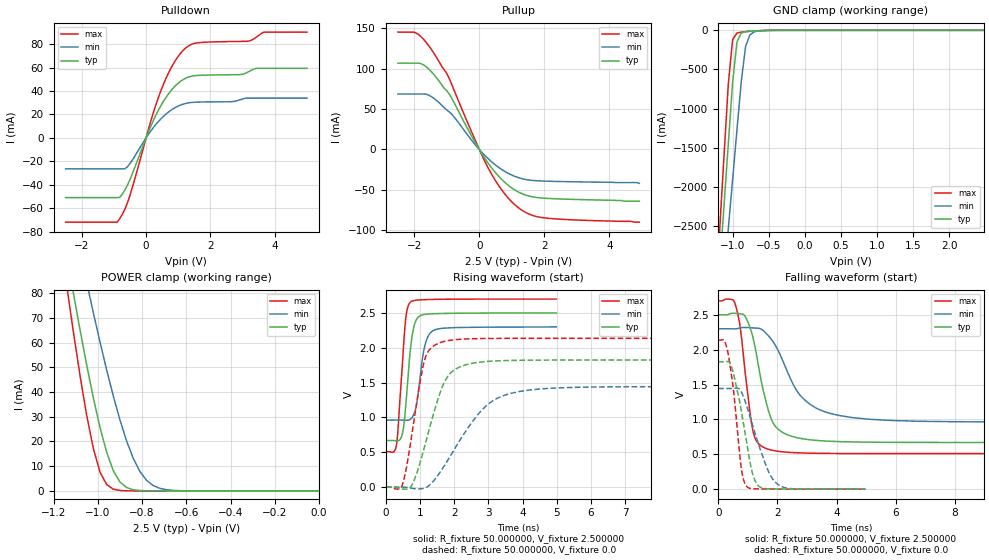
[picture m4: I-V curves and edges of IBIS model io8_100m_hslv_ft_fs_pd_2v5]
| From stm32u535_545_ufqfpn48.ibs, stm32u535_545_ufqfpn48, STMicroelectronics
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|   Model io8_100m_hslv_ft_fs_pd_2v5
[Model]  io8_100m_hslv_ft_fs_pd_2v5
Model_type I/O
Polarity   Non-Inverting
Enable   Active-Low
Vinl =   0.750000V
Vinh =   1.750000V
Vmeas =  1.250000V
Cref =   50.000000pF
Rref =   100.000000M
Vref =   0.0V
C_comp   3.340900pF   3.338500pF   3.380300pF
[Temperature Range]   25.000000   0.140000k   -40.000000
[Pullup Reference]   2.500000V   2.300000V   2.700000V
[Pulldown Reference]   0.0V   0.0V   0.0V
[POWER Clamp Reference]   2.500000V   2.300000V   2.700000V
[GND Clamp Reference]   0.0V   0.0V   0.0V
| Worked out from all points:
|   slope of the pulldown table from 0 to 0.375 V, typ, clamps not added: 16.1 ohm
|   slope of the pullup table from 0 to 0.375 V, typ, clamps not added: 16.6 ohm
|   GND clamp passes 1 mA (typ) near -0.50 V on its own axis
|   POWER clamp passes 1 mA (typ) near -0.86 V on its own axis
|   rising waveform, R_fixture 50.000000, V_fixture 2.500000: 20-80 % time 200ps typ, 231ps min, 180ps max; typ from 0.67 V to 2.5 V
|   rising waveform, R_fixture 50.000000, V_fixture 0.0: 20-80 % time 660ps typ, 1.22ns min, 424ps max; typ from 0 V to 1.82 V
|   falling waveform, R_fixture 50.000000, V_fixture 2.500000: 20-80 % time 569ps typ, 1.09ns min, 362ps max; typ from 2.5 V to 0.67 V
|   falling waveform, R_fixture 50.000000, V_fixture 0.0: 20-80 % time 467ps typ, 671ps min, 321ps max; typ from 1.82 V to 0 V
[Pulldown]
|Voltage   I(typ)   I(min)   I(max)
-2.5V     -51.01mA   -26.45mA   -72.04mA
-900mV    -51.01mA   -26.45mA   -72.04mA
-820mV    -50.89mA   -26.45mA   -69.09mA
-500mV    -35.59mA   -21.93mA   -49.09mA
140mV     9.489mA    5.639mA    13.76mA
460mV     27.5mA     16.25mA    40.22mA
860mV     43.07mA    25.18mA    63.88mA
1.26V     51.38mA    29.65mA    77.49mA
1.66V     53.45mA    30.63mA    81.42mA
3.18V     56.44mA    34.01mA    82.68mA
3.66V     59.44mA    34.01mA    90.42mA
5V        59.44mA    34.01mA    90.42mA
[Pullup]
|Voltage   I(typ)   I(min)   I(max)
-2.5V     106.7mA    68.56mA    145.2mA
-1.96V    106.7mA    68.56mA    144.4mA
-1.72V    104.8mA    68.56mA    136.6mA
-1.48V    96.52mA    65.55mA    124.2mA
-1V       72.68mA    48.88mA    94.22mA
-120mV    8.307mA    5.657mA    10.97mA
280mV     -17.4mA    -11.68mA   -23.32mA
680mV     -36.72mA   -24.56mA   -49.54mA
1.16V     -51.75mA   -34.32mA   -70.71mA
1.56V     -58mA      -38.01mA   -80.45mA
1.96V     -60.18mA   -39.11mA   -84.44mA
4.92V     -64mA      -42mA      -90mA
[GND_clamp]
|Voltage   I(typ)   I(min)   I(max)
-2.5V     -9.446A    -9.524A    -9.146A
-1.18V    -3.045A    -3.8A      -2.552A
-1.12V    -2.248A    -3.166A    -1.614A
-1.06V    -1.452A    -2.533A    -685.4mA
-1V       -665mA     -1.901A    -117.9mA
-940mV    -148mA     -1.272A    -34.34mA
-880mV    -35.14mA   -651.5mA   -22.8mA
-820mV    -16.02mA   -203.9mA   -17.08mA
-760mV    -10.47mA   -56.89mA   -12.28mA
-700mV    -7.079mA   -18.53mA   -8.16mA
-400mV    -112.4uA   -382.5uA   -53.84uA
2.48V     63.1uA     48.03uA    77.39uA
[POWER_clamp]
|Voltage   I(typ)   I(min)   I(max)
-2.49V    881mA      773.1mA    1.07A
-1.14V    95.25mA    122.7mA    82.82mA
-1.11V    79.9mA     109.7mA    64.14mA
-1.05V    50.87mA    84.26mA    30.57mA
-1.02V    37.63mA    72.04mA    17.17mA
-990mV    25.71mA    60.25mA    7.621mA
-930mV    8.217mA    38.43mA    713.9uA
-900mV    3.624mA    28.77mA    182.8uA
-840mV    490.7uA    13.24mA    11.35uA
-780mV    56.55uA    4.324mA    699nA
-660mV    716.5nA    226uA      9.775nA
0V        0A         19.49nA    0A
[Ramp]
| variable   typ   min   max
dV/dt_r  1.09464/0.65908n   0.86550/1.21773n   1.28148/0.42322n
dV/dt_f  1.09787/0.56785n   0.80201/1.08800n   1.31323/0.36140n
R_load = 50.000000
[Rising Waveform]
R_fixture= 50.000000
V_fixture= 2.500000
V_fixture_min= 2.300000
V_fixture_max= 2.700000
|time   V(typ)   V(min)   V(max)
0s        669.5mV    962.5mV    510.4mV
310.3ps   664.1mV    962.9mV    606.2mV
510.5ps   833.7mV    961.8mV    1.977V
600.6ps   1.282V     959.3mV    2.489V
720.7ps   1.991V     975.8mV    2.656V
800.8ps   2.257V     1.028V     2.676V
910.9ps   2.417V     1.229V     2.684V
1.121ns   2.478V     1.988V     2.69V
1.381ns   2.488V     2.246V     2.694V
4.985ns   2.499V     2.299V     2.699V
[Rising Waveform]
R_fixture= 50.000000
V_fixture= 0.0
V_fixture_min= 0.0
V_fixture_max= 0.0
|time   V(typ)   V(min)   V(max)
0s        -172.2uV   -49.94uV   -144.6uV
440.4ps   -21.98mV   -195.2uV   -12.05mV
560.6ps   -29.37mV   -1.621mV   181.7mV
760.8ps   28.65mV    -16.98mV   756.8mV
1.161ns   634.5mV    -10.07mV   1.869V
1.762ns   1.551V     346.1mV    2.097V
2.162ns   1.725V     670mV      2.122V
2.963ns   1.804V     1.179V     2.134V
4.244ns   1.823V     1.396V     2.135V
19.94ns   1.825V     1.442V     2.136V
[Falling Waveform]
R_fixture= 50.000000
V_fixture= 2.500000
V_fixture_min= 2.300000
V_fixture_max= 2.700000
|time   V(typ)   V(min)   V(max)
0s        2.499V     2.299V     2.699V
560.6ps   2.521V     2.298V     2.671V
720.7ps   2.515V     2.309V     2.384V
920.9ps   2.47V      2.317V     1.633V
1.121ns   2.257V     2.313V     956.9mV
1.241ns   2.045V     2.31V      735.8mV
1.762ns   1.04V      2.166V     564mV
2.843ns   722.8mV    1.311V     518.9mV
4.444ns   677.7mV    1.031V     511.2mV
19.94ns   669.5mV    962.5mV    510.4mV
[Falling Waveform]
R_fixture= 50.000000
V_fixture= 0.0
V_fixture_min= 0.0
V_fixture_max= 0.0
|time   V(typ)   V(min)   V(max)
0s        1.825V     1.442V     2.136V
190.2ps   1.824V     1.443V     2.137V
330.3ps   1.831V     1.443V     1.952V
510.5ps   1.665V     1.444V     1.441V
780.8ps   1.122V     1.394V     298.5mV
971ps     642.5mV    1.182V     35.85mV
1.291ns   84.27mV    737.8mV    4.163mV
1.702ns   5.349mV    250.3mV    2.075mV
2.042ns   2.912mV    60.29mV    1.196mV
4.985ns   -172.2uV   -49.94uV   -144.6uV
